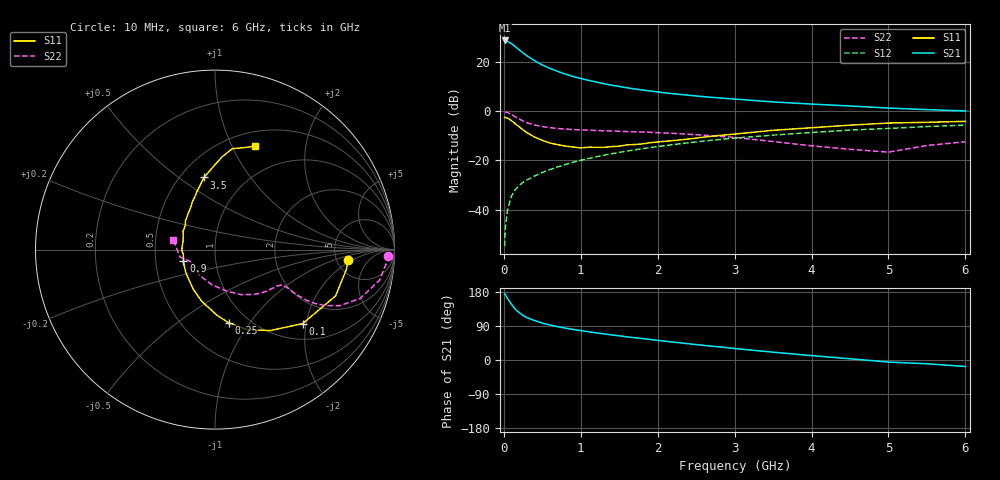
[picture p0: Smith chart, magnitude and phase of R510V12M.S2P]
! SIEMENS Small Signal Semiconductors
! BFR183
! Si NPN RF Bipolar Junction Transistor in SOT23
! VCE = 10 V  IC = 12 mA
! Common Emitter S-Parameters:  May  1996
# GHz  S  MA  R  50
!  f  S11  S21  S12  S22
! GHz  MAG  ANG  MAG  ANG  MAG  ANG  MAG  ANG
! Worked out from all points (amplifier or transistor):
!   36 points, 10 MHz to 6 GHz, reference 50 ohm
!   highest |S21| = 28.7 dB at 10 MHz (marker M1)
!   |S21| within 3 dB of that: start of sweep to 167.9 MHz
!   unconditionally stable (mu >= 1): 778.1 MHz to 2.666 GHz
!   at 250 MHz: K = 0.65, MSG = 26.3 dB, |S12| = -28.9 dB
!   at 1.4 GHz: K = 1.05, MAG = 12.6 dB, |S12| = -17.3 dB
!   at 6 GHz: K = 0.89, MSG = 2.9 dB, |S12| = -5.7 dB
!   S11 on the Smith chart (normalised r, x): 10 MHz: 6.44, -1.62; 100 MHz: 1.37, -1.91; 250 MHz: 0.81, -0.80; 900 MHz: 0.70, -0.09; 3.5 GHz: 0.65, +0.62; 6 GHz: 0.66, +1.23
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0.01  0.7456 -4.3  27.22 175.6  0.0018 85.2  0.9666 -2.0
0.02  0.7398 -8.7  27.13 171.9  0.0044 74.8  0.9589 -4.3
0.05  0.7198 -21.0  26.08 161.9  0.0102 78.1  0.9328 -10.5
0.1  0.639 -40.2  23.48 146.7  0.0189 73.6  0.8535 -18.6
0.15  0.5465 -55.6  20.32 133.8  0.0255 67.4  0.7622 -24.2
0.2  0.4804 -68.3  17.53 124.9  0.0309 64.8  0.6901 -26.9
0.25  0.4145 -79.5  15.18 117.5  0.0357 64.3  0.6283 -28.4
0.3  0.3653 -88.4  13.3 111.8  0.0399 64.0  0.5811 -29.0
0.4  0.297 -104.5  10.55 104.1  0.0481 64.5  0.5212 -28.9
0.5  0.2539 -117.9  8.643 97.4  0.0564 65.2  0.4837 -28.4
0.6  0.2244 -129.6  7.364 92.3  0.065 65.8  0.4594 -27.9
0.7  0.2079 -141.1  6.405 87.9  0.0733 66.6  0.443 -27.7
0.9  0.1867 -160.4  5.048 80.7  0.0913 66.1  0.4217 -27.9
1.1  0.1848 -178.3  4.215 74.6  0.1087 66.0  0.4091 -29.4
1.3  0.1837 166.0  3.599 69.0  0.127 65.0  0.3982 -30.9
1.6  0.2059 150.2  2.974 61.1  0.154 62.9  0.3828 -34.4
2.2  0.2513 126.3  2.249 47.3  0.2087 57.7  0.353 -43.3
3.5  0.4067 98.6  1.536 20.6  0.3245 42.8  0.2407 -74.0
4.5  0.5177 85.7  1.268 3.3  0.411 31.0  0.1671 -121.2
5  0.5712 80.2  1.153 -5.4  0.444 23.7  0.1463 -151.1
5.5  0.592 73.7  1.07 -10.0  0.484 19.6  0.1998 -168.2
6  0.618 68.9  1.008 -17.1  0.52 12.3  0.2379 167.1
